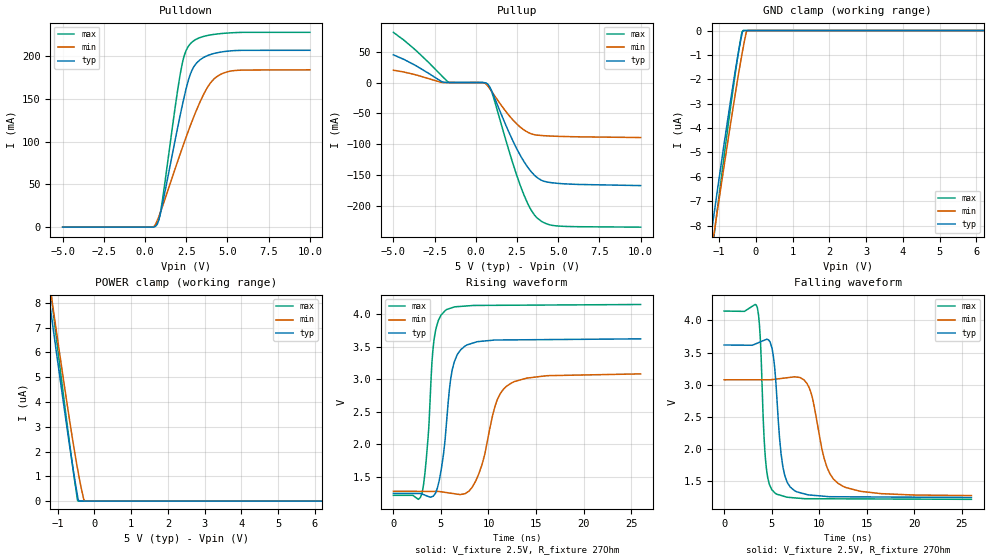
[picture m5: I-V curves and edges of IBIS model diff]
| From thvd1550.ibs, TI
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|   diff Model
[Model]   diff
Model_type   I/O
Polarity   Non-Inverting
Enable   Active-High
Vinl = 0.5
Vinh = 4.5
Vmeas = 2.5
Vref = 2.5
Cref = 2pF
Rref = 27
|   typ   min   max
C_comp   1.87792E-11   1.86058E-11   1.88619E-11
| Where Nom  PVT is Nominal Process, 5V, 27C
|   Fast PVT is Strong Process,  5.5V, -40C
|   Slow PVT is Weak Process,   4.5, 150C
[Voltage Range]   5   4.5   5.5
|Junction Temperature
[Temperature Range]   27   150   -40
[Pullup Reference]   5   4.5   5.5
[Pulldown Reference]   0   0   0
[Power Clamp Reference]   5   4.5   5.5
[GND Clamp Reference]   0   0   0
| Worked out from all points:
|   slope of the pulldown table from 0 to 0.75 V, typ, clamps not added: 188 ohm
|   slope of the pullup table from 0 to 0.75 V, typ, clamps not added: 218 ohm
|   falling waveform, V_fixture 2.5V, R_fixture 27Ohm: 20-80 % time 799ps typ, 1.66ns min, 519ps max; typ from 3.62 V to 1.25 V
|   rising waveform, V_fixture 2.5V, R_fixture 27Ohm: 20-80 % time 1.05ns typ, 1.84ns min, 763ps max; typ from 1.25 V to 3.62 V
[Pulldown]
|   Voltage   I(typ)   I(min)   I(max)
-5V       -31.71uA   -27.3uA    -35.51uA
385mV     -11.23uA   26.35uA    -16.77uA
670mV     1.686mA    4.655mA    2.662mA
865mV     10.68mA    13.84mA    11.47mA
985mV     20.65mA    20.28mA    23.04mA
1.87V     106.3mA    70.94mA    146.3mA
2.245V    141.4mA    92.04mA    190.6mA
2.5V      162.7mA    105.9mA    207.3mA
2.92V     186.6mA    127.5mA    217.8mA
3.82V     201.2mA    164.8mA    224.6mA
4.705V    205.4mA    180mA      226.9mA
10V       207.1mA    184.2mA    228.2mA
[GND Clamp]
|   Voltage   I(typ)   I(min)   I(max)
-5V       -51.33uA   -49.63uA   -57.43uA
-1.25V    -8.717uA   -9.457uA   -9.764uA
-1.04V    -6.479uA   -7.319uA   -7.232uA
-815mV    -4.143uA   -5.063uA   -4.583uA
-575mV    -1.793uA   -2.735uA   -1.911uA
-485mV    -988.9nA   -1.903uA   -998.1nA
-410mV    -379.7nA   -1.239uA   -313.3nA
-380mV    -157.6nA   -983.7nA   -68.67nA
-350mV    -26.35nA   -736.7nA   0A
-260mV    0A         -60.03nA   0A
-230mV    0A         0A         0A
10V       0A         0A         0A
[Pullup]
|   Voltage   I(typ)   I(min)   I(max)
-5V       44.84mA    20.01mA    81.22mA
-3.575V   26.37mA    11.98mA    50.56mA
-1.7V     37.7uA     27.73uA    1.39mA
415mV     9.164uA    -58.8uA    22.5uA
730mV     -2.694mA   -5.667mA   -3.998mA
1.03V     -17.85mA   -16.89mA   -20.19mA
2.08V     -84.49mA   -55.22mA   -116.2mA
2.755V    -120.3mA   -73.26mA   -170.3mA
3.265V    -141mA     -81.77mA   -201.8mA
3.76V     -154.4mA   -85.09mA   -219.8mA
5.02V     -163.1mA   -86.95mA   -232mA
10V       -166.6mA   -88.88mA   -233.8mA
[POWER Clamp]
|   Voltage   I(typ)   I(min)   I(max)
-5V       52.07uA    51.03uA    57.36uA
-1.25V    8.356uA    9.1uA      9.212uA
-1.1V     6.725uA    7.542uA    7.378uA
-845mV    4uA        4.941uA    4.312uA
-695mV    2.446uA    3.459uA    2.565uA
-560mV    1.114uA    2.188uA    1.068uA
-455mV    173.4nA    1.281uA    15.25nA
-440mV    51.54nA    1.158uA    7.626nA
-410mV    0A         920.7nA    0A
-290mV    0A         75.9nA     0A
-260mV    0A         0A         0A
10V       0A         0A         0A
[Ramp]
R_load = 27
|   typ   min   max
dV/dt_r   1.42112/1.04505e-09   1.07901/1.82149e-09   1.75413/7.60156e-10
dV/dt_f   1.42095/7.95626e-10   1.07878/1.64818e-09   1.75408/5.17683e-10
[Falling Waveform]
V_fixture = 2.5V
V_fixture_min = 2.25V
V_fixture_max = 2.75V
R_fixture = 27Ohm
C_fixture = 0F
|   Time   V(typ)   V(min)   V(max)
0s        3.617V     3.076V     4.144V
3.481ns   3.645V     3.076V     4.201V
3.79ns    3.664V     3.076V     3.752V
4.388ns   3.701V     3.076V     1.779V
5.358ns   3.192V     3.086V     1.317V
6.158ns   1.743V     3.1V       1.273V
7.407ns   1.355V     3.123V     1.243V
8.952ns   1.288V     2.95V      1.23V
11.94ns   1.26V      1.473V     1.228V
26ns      1.249V     1.278V     1.22V
[Rising Waveform]
V_fixture = 2.5V
V_fixture_min = 2.25V
V_fixture_max = 2.75V
R_fixture = 27Ohm
C_fixture = 0F
|   Time   V(typ)   V(min)   V(max)
0s        1.25V      1.283V     1.221V
2.993ns   1.242V     1.282V     1.243V
3.638ns   1.205V     1.281V     2.089V
4.25ns    1.22V      1.281V     3.575V
5.447ns   2.089V     1.266V     4.051V
6.207ns   3.155V     1.25V      4.097V
7.762ns   3.526V     1.267V     4.123V
8.997ns   3.577V     1.556V     4.13V
11.94ns   3.602V     2.898V     4.133V
26ns      3.618V     3.081V     4.144V
